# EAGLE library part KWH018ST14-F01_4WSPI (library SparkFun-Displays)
Fomike KWH018ST14-F01 TFT LCD Module Using 4WSPI Interface 128 x 160 pixel 18-bit color depth LCD module with LED backlight. This part uses the 4WSPI interface, though several other interface options are broken out in the FPC cable. Use the other corresponding devices for 3WSPI, and 8/9/16/18 bit parallel. Note: PROD_ID corresponds to the connector and the second ID (PROD_ID1 = LCD-14196) corresponds to the actual module Variants: Bottom - For use with bottom-contact FPC connectors Top - For use with top-contact FPC connectors SparkFun Products:
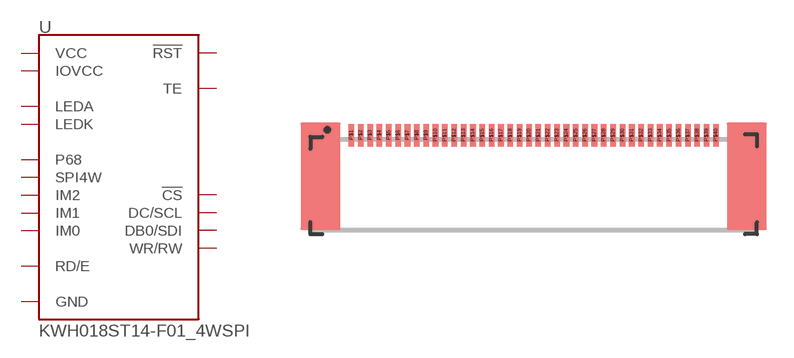
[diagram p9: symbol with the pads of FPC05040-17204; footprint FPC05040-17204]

Designator prefix U

## KWH018ST14-F01_4WSPI-TOP (PROD_ID: CONN-14082; PROD_ID1: LCD-14196)  [FPC05040-17204]
P$1  GND
P$6  GND
P$7  IM0
P$8  IM1
P$9  IM2
P$10  P68
P$11  SPI4W
P$12  !CS
P$13  DC/SCL
P$14  WR/RW
P$15  RD/E
P$16  DB0/SDI
P$17  GND
P$18  GND
P$19  GND
P$20  GND
P$21  GND
P$22  GND
P$23  GND
P$24  GND
P$25  GND
P$26  GND
P$27  GND
P$28  GND
P$29  GND
P$30  GND
P$31  GND
P$32  GND
P$33  GND
P$34  TE
P$35  IOVCC
P$36  VCC
P$37  !RST
P$38  GND
P$39  LEDK
P$40  LEDA

## KWH018ST14-F01_4WSPI-BOTTOM (PROD_ID: CONN-14082; PROD_ID1: LCD-14196)  [FPC05040-17204]
P$1  LEDA
P$2  LEDK
P$3  GND
P$4  !RST
P$5  VCC
P$6  IOVCC
P$7  TE
P$8  GND
P$9  GND
P$10  GND
P$11  GND
P$12  GND
P$13  GND
P$14  GND
P$15  GND
P$16  GND
P$17  GND
P$18  GND
P$19  GND
P$20  GND
P$21  GND
P$22  GND
P$23  GND
P$24  GND
P$25  DB0/SDI
P$26  RD/E
P$27  WR/RW
P$28  DC/SCL
P$29  !CS
P$30  SPI4W
P$31  P68
P$32  IM2
P$33  IM1
P$34  IM0
P$35  GND
P$40  GND

## Footprint FPC05040-17204 (pad centres in mm)
FPC05040 - This is a 0.5mm pitch FPC connector with 40 positions Specifications: Pin count: 40 Pin pitch: 0.5mm Area: 20mm x 5mm Datasheet referenced for footprint Example device(s):
smd 0.3 x 1.2: P$1 -9.75,0.6; P$2 -9.25,0.6; P$3 -8.75,0.6; P$4 -8.25,0.6; P$5 -7.75,0.6; P$6 -7.25,0.6; P$7 -6.75,0.6; P$8 -6.25,0.6; P$9 -5.75,0.6; P$10 -5.25,0.6; P$11 -4.75,0.6; P$12 -4.25,0.6; P$13 -3.75,0.6; P$14 -3.25,0.6; P$15 -2.75,0.6; P$16 -2.25,0.6; P$17 -1.75,0.6; P$18 -1.25,0.6; P$19 -0.75,0.6; P$20 -0.25,0.6; P$21 0.25,0.6; P$22 0.75,0.6; P$23 1.25,0.6; P$24 1.75,0.6; P$25 2.25,0.6; P$26 2.75,0.6; P$27 3.25,0.6; P$28 3.75,0.6; P$29 4.25,0.6; P$30 4.75,0.6; P$31 5.25,0.6; P$32 5.75,0.6; P$33 6.25,0.6; P$34 6.75,0.6; P$35 7.25,0.6; P$36 7.75,0.6; P$37 8.25,0.6; P$38 8.75,0.6; P$39 9.25,0.6; P$40 9.75,0.6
